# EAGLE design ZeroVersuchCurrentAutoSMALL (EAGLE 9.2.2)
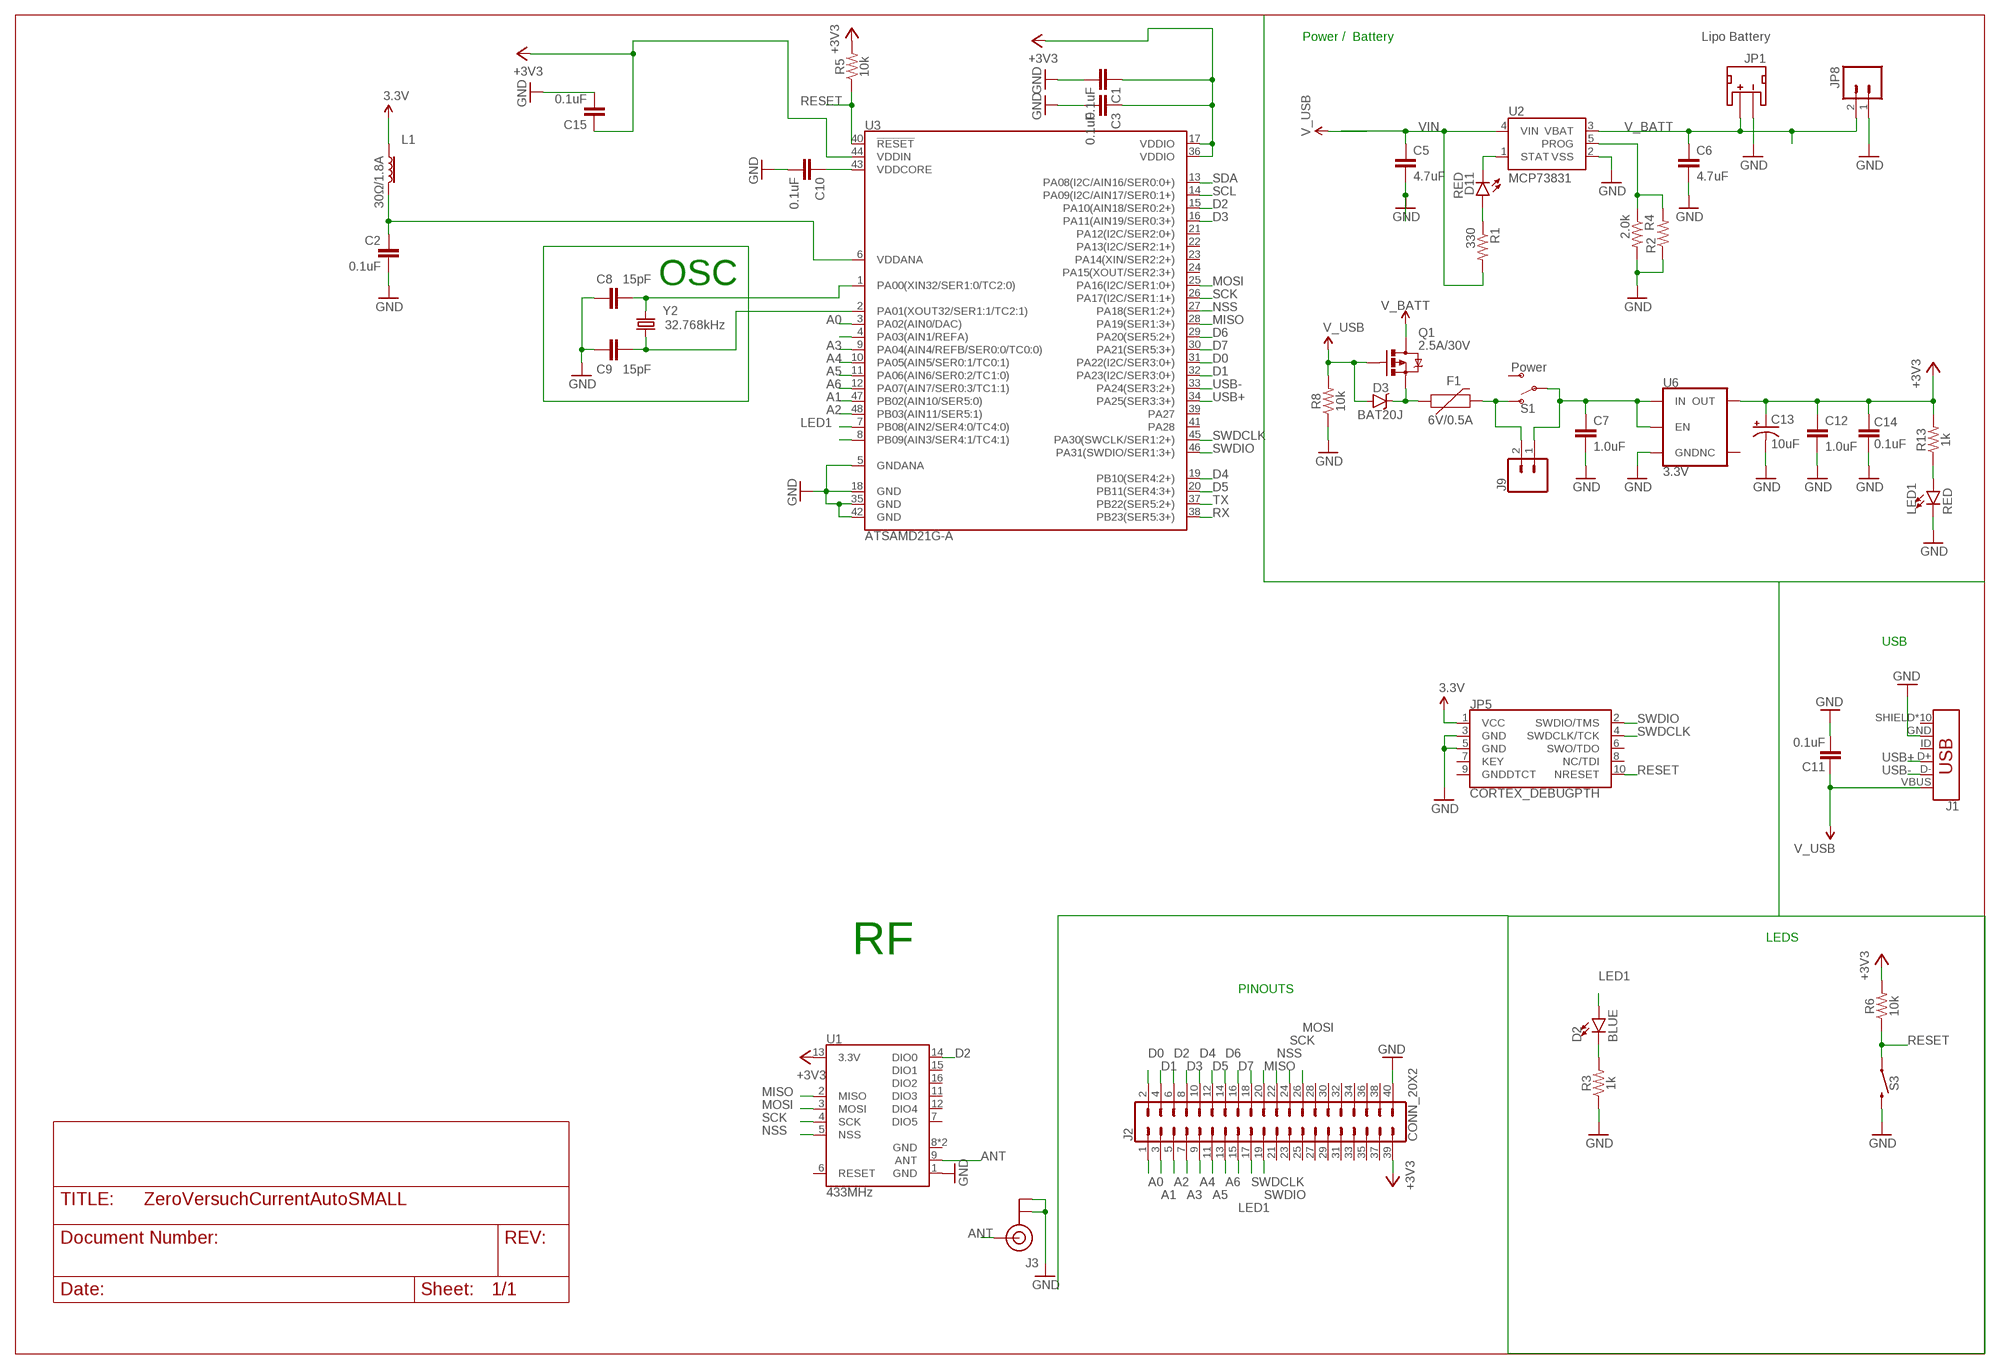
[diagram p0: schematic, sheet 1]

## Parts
C1  0.1uF  0.1UF-KIT-EZ-50V-20%  [CAP-PTH-SMALL-KIT]
C2  0.1uF  0.1UF-KIT-EZ-50V-20%  [CAP-PTH-SMALL-KIT]
C3  0.1uF  0.1UF-KIT-EZ-50V-20%  [CAP-PTH-SMALL-KIT]
C5  4.7uF  4.7UF-1206-16V-(+80/-20%)  [1206]
C6  4.7uF  4.7UF-1206-16V-(+80/-20%)  [1206]
C7  1.0uF  1.0UF-0603-16V-10%  [0603]
C8  15pF  15PF-0603-50V-5%  [0603]
C9  15pF  15PF-0603-50V-5%  [0603]
C10  0.1uF  0.1UF-KIT-EZ-50V-20%  [CAP-PTH-SMALL-KIT]
C11  0.1uF  0.1UF-KIT-EZ-50V-20%  [CAP-PTH-SMALL-KIT]
C12  1.0uF  1.0UF-0603-16V-10%  [0603]
C13  10uF  10UF-POLAR-RADIAL-2.5MM-KIT-25V-20%  [CPOL-RADIAL-2.5MM-5MM-KIT]
C14  0.1uF  0.1UF-KIT-EZ-50V-20%  [CAP-PTH-SMALL-KIT]
C15  0.1uF  0.1UF-KIT-EZ-50V-20%  [CAP-PTH-SMALL-KIT]
D2  BLUE  LED-BLUE1206  [LED-1206]
D3  BAT20J  DIODE-SCHOTTKY-BAT20J  [SOD-323]
D11  RED  LED-RED1206  [LED-1206]
F1  6V/0.5A  PPTC_HALF-AMP  [1206]
J1  USB_MICRO-B_HALF_PTH_MILL  [USB-MICROB-PTH-MILL]
J2  CONN_20X2  [2X20]
J3  U.FL  [U.FL]
J9  External On/Off  CONN_021X02_NO_SILK  [1X02_NO_SILK]
JP1  JST  JST_2MM_MALE  [JST-2-SMD@1]
JP5  CORTEX_DEBUGPTH  [2X5-PTH-1.27MM]
JP8  M02PTH  [1X02@1]
L1  30Ω/1.8A  FERRITE_BEAD-0603  [0603]
LED1  RED  LED-RED1206  [LED-1206]
Q1  2.5A/30V  MOSFET-PCHANNELDMG2307L  [SOT23-3]
R1  330  330OHM-HORIZ-1/10W-5%  [AXIAL-0.3]
R2  RESISTORPTH-1/4W-VERT-KIT  [AXIAL-0.1EZ]
R3  1k  1KOHM-HORIZ-1/4W-5%  [AXIAL-0.3]
R4  2.0k  2.0KOHM1/10W5%(0603)  [0603-RES]
R5  10k  10KOHM-HORIZ-1/4W-5%  [AXIAL-0.3]
R6  10k  10KOHM-HORIZ-1/4W-5%  [AXIAL-0.3]
R8  10k  10KOHM-HORIZ-1/4W-5%  [AXIAL-0.3]
R13  1k  1KOHM-HORIZ-1/4W-5%  [AXIAL-0.3]
S1  Power  SWITCH-SPDT-SMD-RIGHT-ANGLE  [SWITCH_SPST_SMD_A]
S3  MOMENTARY-SWITCH-SPST-SMD-RIGHT-ANGLE  [TACTILE_SWITCH_SMD_RIGHT_ANGLE]
U1  433MHz  RFM69HCW-433  [RFM69HCW-XXXS2]
U2  MCP73831  [SOT23-5]
U3  ATSAMD21G-A  [TQFP-48]
U6  3.3V  V_REG_AP2112K-3.3V  [SOT23-5]
Y2  32.768kHz  CRYSTAL-32.768KHZSMD-3.2X1.5  [CRYSTAL-SMD-3.2X1.5MM]

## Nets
3.3V [vcc]: JP5.1(VCC) L1.1
+3V3: C1.1 C3.1 C12.1 C13.1(+) C14.2 C15.1 J2.39 R5.P$2 R6.P$2 R13.P$2 U1.13(3.3V) U3.17(VDDIO) U3.36(VDDIO) U3.44(VDDIN) U6.5(OUT)
A0: J2.1 U3.3(PA02(AIN0/DAC))
A1: J2.3 U3.47(PB02(AIN10/SER5:0))
A2: J2.5 U3.48(PB03(AIN11/SER5:1))
A3: J2.7 U3.9(PA04(AIN4/REFB/SER0:0/TC0:0))
A4: J2.9 U3.10(PA05(AIN5/SER0:1/TC0:1))
A5: J2.11 U3.11(PA06(AIN6/SER0:2/TC1:0))
A6: J2.13 U3.12(PA07(AIN7/SER0:3/TC1:1))
ANT: J3.FEED(SIGNAL) U1.9(ANT)
D0: J2.2 U3.31(PA22(I2C/SER3:0+))
D1: J2.4 U3.32(PA23(I2C/SER3:0+))
D2: J2.6 U1.14(DIO0) U3.15(PA10(AIN18/SER0:2+))
D3: J2.8 U3.16(PA11(AIN19/SER0:3+))
D4: J2.10 U3.19(PB10(SER4:2+))
D5: J2.12 U3.20(PB11(SER4:3+))
D6: J2.14 U3.29(PA20(SER5:2+))
D7: J2.16 U3.30(PA21(SER5:3+))
GND: C1.2 C2.2 C3.2 C5.2 C6.2 C7.2 C8.1 C9.1 C10.2 C11.1 C12.2 C13.2(-) C14.1 C15.2 J1.GND J2.40 J3.1(GND) J3.2(GND) JP1.1(-) JP5.3(GND) JP5.5(GND) JP8.1 LED1.C R2.P$1 R3.P$1 R4.2 R8.P$1 S3.2 U1.1(GND) U2.2(VSS) U3.5(GNDANA) U3.18(GND) U3.35(GND) U3.42(GND) U6.2(GND)
LED1: D2.A J2.15 U3.7(PB08(AIN2/SER4:0/TC4:0))
MISO: J2.20 U1.2(MISO) U3.28(PA19(SER1:3+))
MOSI: J2.26 U1.3(MOSI) U3.25(PA16(I2C/SER1:0+))
N$1: D2.C R3.P$2
N$2: C10.1 U3.43(VDDCORE)
N$4: D11.A R1.P$1
N$8: C7.1 J9.1 S1.2(P) U6.1(IN) U6.3(EN)
N$9: F1.2 J9.2 S1.1(O)
N$10: C8.2 U3.1(PA00(XIN32/SER1:0/TC2:0)) Y2.P$2
N$11: C9.2 U3.2(PA01(XOUT32/SER1:1/TC2:1)) Y2.P$1
N$14: U3.4(PA03(AIN1/REFA))
N$15: J2.18
N$22: U3.8(PB09(AIN3/SER4:1/TC4:1))
N$38: LED1.A R13.P$1
NSS: J2.22 U1.5(NSS) U3.27(PA18(SER1:2+))
PROG: R2.P$2 R4.1 U2.5(PROG)
RAW [vcc]: D3.C F1.1 Q1.2(S)
RESET: JP5.10(NRESET) R5.P$1 R6.P$1 S3.1 U3.40(!RESET!)
RX: U3.38(PB23(SER5:3+))
SCK: J2.24 U1.4(SCK) U3.26(PA17(I2C/SER1:1+))
SCL: U3.14(PA09(I2C/AIN17/SER0:1+))
SDA: U3.13(PA08(I2C/AIN16/SER0:0+))
STAT: D11.C U2.1(STAT)
SWDCLK: J2.17 JP5.4(SWDCLK/TCK) U3.45(PA30(SWCLK/SER1:2+))
SWDIO: J2.19 JP5.2(SWDIO/TMS) U3.46(PA31(SWDIO/SER1:3+))
TX: U3.37(PB22(SER5:2+))
USB+: J1.D+ U3.34(PA25(SER3:3+))
USB-: J1.D- U3.33(PA24(SER3:2+))
V_BATT: C6.1 JP1.2(+) JP8.2 Q1.3(D) U2.3(VBAT)
V_USB: C11.2 D3.A J1.VBUS Q1.1(G) R8.P$2
VDDANA: C2.1 L1.2 U3.6(VDDANA)
VIN: C5.1 R1.P$2 U2.4(VIN)
Unconnected: J1.ID J1.SHIELD J1.SHIELD2(SHIELD) J1.SHIELD3(SHIELD) J1.SHIELD4(SHIELD) J1.SHIELD5(SHIELD) J1.SHIELD6(SHIELD) J1.SHIELD7(SHIELD) J1.SHIELD8(SHIELD) J1.SHIELD9(SHIELD) J1.SHIELD10(SHIELD) J2.21 J2.23 J2.25 J2.27 J2.28 J2.29 J2.30 J2.31 J2.32 J2.33 J2.34 J2.35 J2.36 J2.37 J2.38 JP1.NC1(PAD1) JP1.NC2(PAD2) JP5.6(SWO/TDO) JP5.7(KEY) JP5.8(NC/TDI) JP5.9(GNDDTCT) S1.3(S) U1.6(RESET) U1.7(DIO5) U1.11(DIO3) U1.12(DIO4) U1.15(DIO1) U1.16(DIO2) U3.21(PA12(I2C/SER2:0+)) U3.22(PA13(I2C/SER2:1+)) U3.23(PA14(XIN/SER2:2+)) U3.24(PA15(XOUT/SER2:3+)) U3.39(PA27) U3.41(PA28) U6.4(NC)

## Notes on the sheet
- Power /  Battery | Lipo Battery
- OSC
- USB
- LEDS
- RF
- PINOUTS

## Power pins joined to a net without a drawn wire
GND: U1.8(GND) U1.10(GND)

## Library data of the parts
C1-C3 C10 C11 C14 C15 = SparkFun-Capacitors:0.1UF: 0.1µF ceramic capacitors; PROD_ID: CAP-08370
C5 C6 = SparkFun-Capacitors:4.7UF: 4.7µF ceramic capacitors; PROD_ID: CAP-10300
C7 C12 = SparkFun-Capacitors:1.0UF: 1µF ceramic capacitors; PROD_ID: CAP-00868
C8 C9 = SparkFun-Capacitors:15PF: 15pF ceramic capacitors; PROD_ID: CAP-07881
C13 = SparkFun-Capacitors:10UF-POLAR: 10.0µF polarized capacitors; PROD_ID: CAP-08440
D2 = SparkFun-LED:LED-BLUE: Blue SMD LED; PROD_ID: DIO-09911
D3 = SparkFun-DiscreteSemi:DIODE-SCHOTTKY: Schottky diodes in SFE's production catalog; PROD_ID: DIO-11623
D11 LED1 = SparkFun-LED:LED-RED: Red SMD LED; PROD_ID: DIO-09912
F1 = SparkFun-Fuses:PPTC: Resettable Fuse PPTC; PROD_ID: RES-08585
J1 = SparkFun-Connectors:USB_MICRO-B: USB Type Micro-B Connector Male/female and PTH/SMT variants SparkFun Products: SparkFun microB USB Breakout SparkFun USB microB Plug Breakout SparkFun ESP8266 Thing; PROD_ID: CONN-13711
J2 = SparkFun-Connectors:CONN_20X2: Multi connection point. Often used as Generic Header-pin footprint for 0.1 inch spaced/style header connections On any of the 0.1 inch spaced packages, you can populate with these: Break Away Headers - Straight (PRT-00116) Break Away Male Headers - Right Angle (PRT-00553) Female Headers (PRT-00115)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
J3 = SparkFun-Connectors:U.FL: SMD Antenna Connector - U.FL 2mm height, 3.0mm x 3.0mm receptacle size. SparkFun Products: SparkFun WiFi Shield - ESP8266 SparkFun ESP8266 Thing SparkFun MiniGen - Pro Mini Signal Generator Shield; PROD_ID: CONN-09193; SF_ID: WRL-09144
J9 = SparkFun-Connectors:CONN_02: Multi connection point. Often used as Generic Header-pin footprint for 0.1 inch spaced/style header connections
JP1 = SparkFun-Connectors:JST_2MM_MALE: Mates to single-cell LiPo batteries. CONN-08352; PROD_ID: CONN-08352
JP5 = samd21-temp:CORTEX_DEBUG: Cortex Debug Connector Datasheet
JP8 = SparkFun-Connectors:M02: Standard 2-pin 0.1" header. Use with
L1 = SparkFun-Coils:FERRITE_BEAD: Ferrite Bead (blocks, cores, rings, chokes, etc.); PROD_ID: NDUC-07859
Q1 = SparkFun-DiscreteSemi:MOSFET-PCHANNEL: Generic PMOSFET IRLML2244 - TRANS-11153 (SOT-23 -20V -4.3A) (1.Gate 2.Source 3.Drain) FQP27P06 - COM-10349 (TO-220 -60V -27A) (1.Gate 2.Source 3.Drain); PROD_ID: TRANS-11308
R1 = SparkFun-Resistors:330OHM: 330Ω resistor; PROD_ID: RES-8371
R2 = SparkFun-Resistors:RESISTOR: Resistor
R3 R13 = SparkFun-Resistors:1KOHM: 1kΩ resistor; PROD_ID: RES-08380
R4 = SparkFun-Resistors:2.0KOHM1/10W5%(0603): RES-08296; PROD_ID: RES-08296
R5 R6 R8 = SparkFun-Resistors:10KOHM: 10kΩ resistor; PROD_ID: RES-09435
S1 = SparkFun-Switches:SWITCH-SPDT: Single Pole, Double Throw (SPDT) Switch Single-pole, double-throw (SPDT) switch. Variant Overview SMD-AYZ0202 Surface Mount DPDT Switch (COM-00597) Used on e.g. LilyPad Arduino USB - ATmega32U4 Board PTH-11.6X4.0MM SPDT Mini Power Switch (COM-00102) Used on e.g. SparkFun Simon Says - Through-Hole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; PROD_ID: SWCH-10651; SF_SKU: COM-10860
S3 = SparkFun-Switches:MOMENTARY-SWITCH-SPST: Momentary Switch (Pushbutton) - SPST; PROD_ID: COMP-12265
U1 = SparkFun-RF:RFM69H: Hope RF RFM69H ISM Transceiver Module The RFM69H is a transceiver module capable of operation over a wide frequency range, including the 315,433,868 and 915MHz license-free ISM (Industry Scientific and Medical) frequency bands. All major RF communication parameters are programmable and most of them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; PROD_ID: IC-12053
U2 = SparkFun-PowerIC:MCP73831: Miniature single cell, fully integrated Li-Ion, Li-polymer charge management controller http://ww1.microchip.com/downloads/en/DeviceDoc/21984a.pdf IC-09995; PROD_ID: IC-09995
U3 = SparkFun-IC-Microcontroller:ATSAMD21G: Atmel SAMD21G SMART ARM-Based Microcontroller The Atmel ® | SMART ™ SAM D21 is a series of low-power microcontrollers using the 32-bit ARM ® Cortex ® -M0+ processor, and ranging from 32- to 64-pins with up to 256KB Flash and 32KB of SRAM. The SAM D21 devices operate at a maximum frequency of 48MHz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; PROD_ID: IC-13064
U6 = SparkFun-IC-Power:V_REG_AP2112: AP2112 - 600mA CMOS LDO Regulator w/ Enable The AP2112 is CMOS process low dropout linear regulator with enable function, the regulator delivers a guaranteed 600mA (min.) continuous load current. Features Output Voltage Accuracy: ±1.5% Output Current: 600mA (Min.) Foldback Short Current Protection: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; PROD_ID: VREG-12457
Y2 = SparkFun-Clocks:CRYSTAL-32.768KHZ: 32.768kHz Crystal; PROD_ID: XTAL-13062

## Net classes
0 default: width 0.01 mm, drill 0.02 mm, clearance 0.006 mm
1 vcc: width 0.01 mm, drill 0.02 mm, clearance 0.006 mm to class 0

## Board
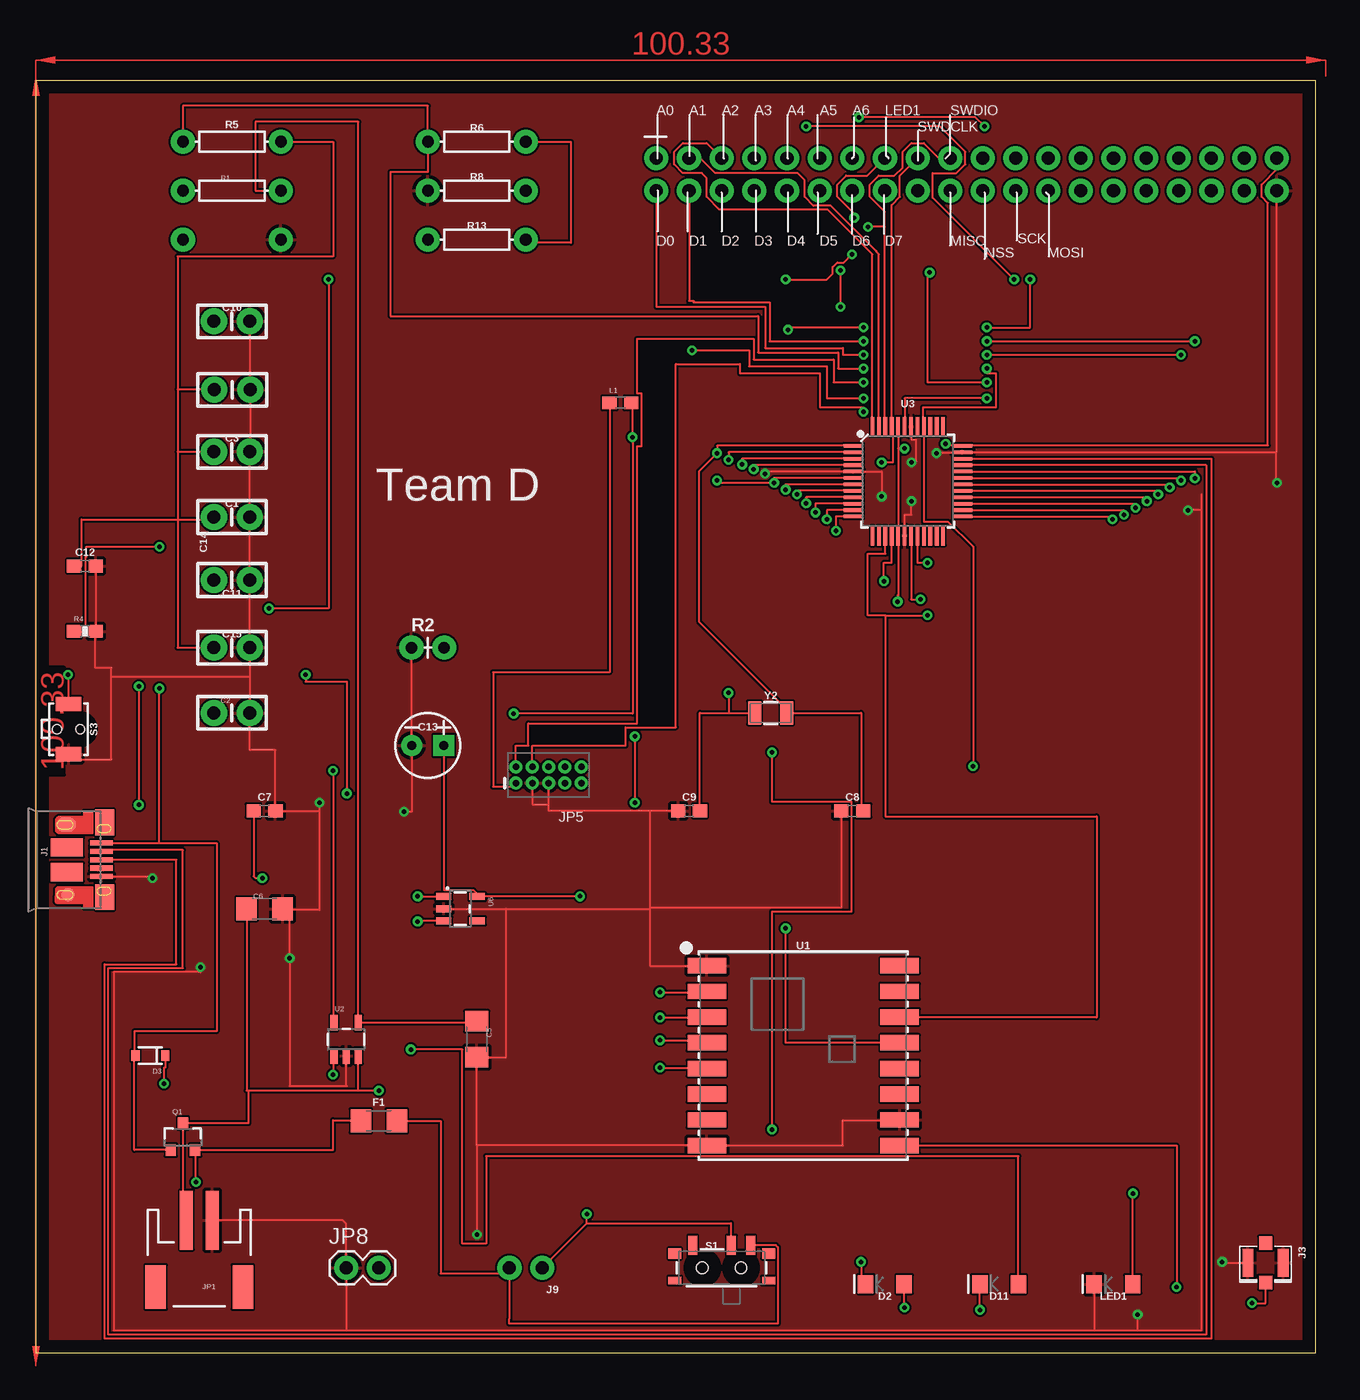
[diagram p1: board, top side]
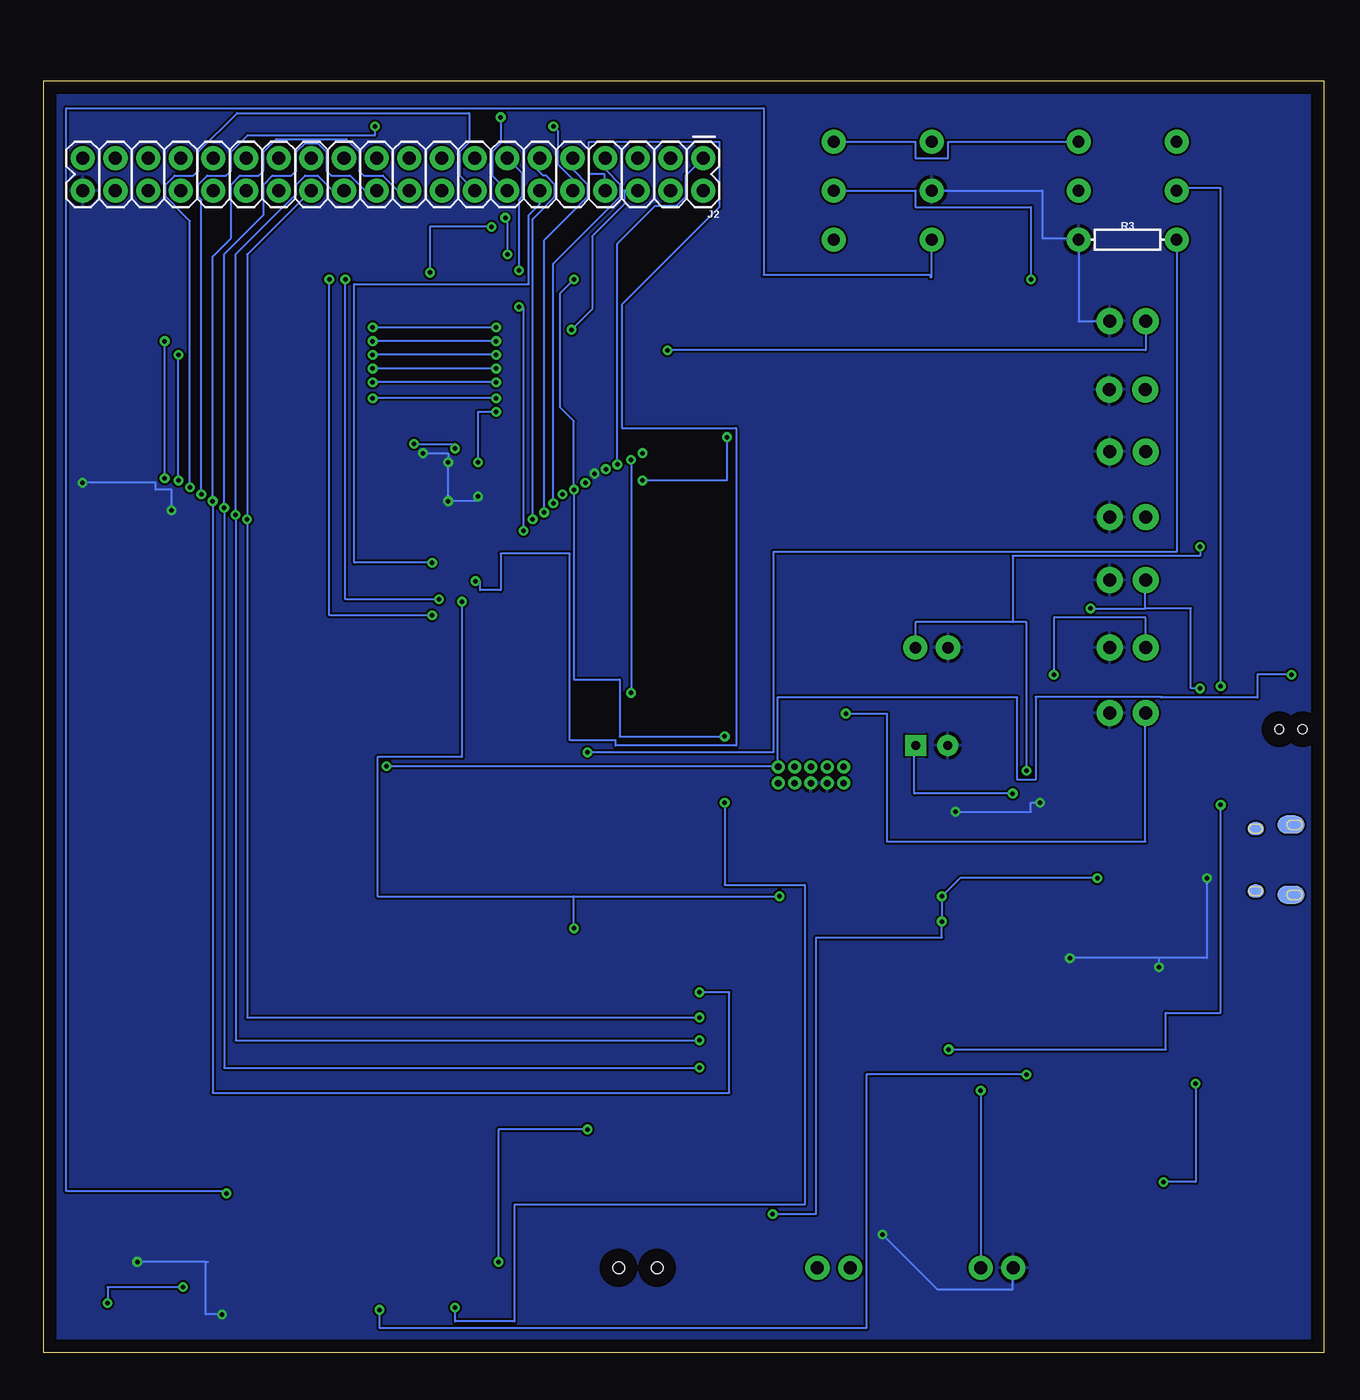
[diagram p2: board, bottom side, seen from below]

Size 99.55 x 98.98 mm. Coordinates in mm from the lower left corner, seen from the top.
Outline: 0,0 99.55,0 99.55,98.98 0,98.98 0,0
Copper layers (1*16): Top 0.035mm / dielectric 1.5mm / Bottom 0.035mm
Design rules "default": minimum track width 6mil, minimum drill 0.35mm, track to track 6mil, track to pad 6mil, pad to pad 6mil, via to via 6mil, smd to smd 6mil, copper to edge 40mil, drill to drill 6mil, minimum pad ring 10mil, minimum via ring 8mil, stop-mask expansion 4mil, vias tented up to drill 0mil, thermal gap 10mil

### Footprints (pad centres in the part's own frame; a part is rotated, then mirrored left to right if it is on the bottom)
CAP-PTH-SMALL-KIT = drill 1.016 pad 2.032: 1 -1.397,0; 2 1.397,0
1206 = smd 1.6 x 1.8: 1 -1.4,0; 2 1.4,0
0603 = smd 1.1 x 1: 1 -0.85,0; 2 0.85,0
CPOL-RADIAL-2.5MM-5MM-KIT = drill 0.7 pad 1.651 square: 1 1.25,0 | drill 0.7 pad 1.651: 2 -1.25,0
LED-1206 = smd 1.2 x 1.4: A -1.5,0; C 1.5,0
SOD-323 = smd 0.63 x 0.83: A 1.15,0; C -1.15,0
USB-MICROB-PTH-MILL = smd 0.4 x 1.75: D+ 0,0; D- -0.65,0; GND 1.3,0; ID 0.65,0; VBUS -1.3,0 | smd 2 x 1.46: SHIELD -2.9,0.275; SHIELD2 2.9,0.275 | smd 1.425 x 2.5: SHIELD3 -0.963,-2.675; SHIELD4 0.963,-2.675 | smd 1.4 x 2.1 bottom: SHIELD5 -2.731,-2.531; SHIELD7 2.729,-2.531 | smd 1 x 1: SHIELD6 2.7,-2.575 | smd 1.1 x 1.5: SHIELD8 -2.731,-2.731 | smd 1 x 1.3 bottom: SHIELD9 -2.43,0.195; SHIELD10 2.43,0.195
2X20 = drill 1.016 pad 1.88: 1 0,0; 2 0,2.54; 3 2.54,0; 4 2.54,2.54; 5 5.08,0; 6 5.08,2.54; 7 7.62,0; 8 7.62,2.54; 9 10.16,0; 10 10.16,2.54; 11 12.7,0; 12 12.7,2.54; 13 15.24,0; 14 15.24,2.54; 15 17.78,0; 16 17.78,2.54; 17 20.32,0; 18 20.32,2.54; 19 22.86,0; 20 22.86,2.54; 21 25.4,0; 22 25.4,2.54; 23 27.94,0; 24 27.94,2.54; 25 30.48,0; 26 30.48,2.54; 27 33.02,0; 28 33.02,2.54; 29 35.56,0; 30 35.56,2.54; 31 38.1,0; 32 38.1,2.54; 33 40.64,0; 34 40.64,2.54; 35 43.18,0; 36 43.18,2.54; 37 45.72,0; 38 45.72,2.54; 39 48.26,0; 40 48.26,2.54
U.FL = smd 2.2 x 0.85: 1 0,1.375; 2 0,-1.375 | smd 1.05 x 1: FEED 1.525,0; NC -1.525,0
1X02_NO_SILK = drill 1.016 pad 1.88: 1 0,0; 2 2.54,0
JST-2-SMD@1 = smd 1 x 4.6: 1 -1,-3.7; 2 1,-3.7 | smd 1.6 x 3.4: NC1 -3.4,1.5; NC2 3.4,1.5
2X5-PTH-1.27MM = drill 0.508 pad 1: 1 -2.54,-0.635; 2 -2.54,0.635; 3 -1.27,-0.635; 4 -1.27,0.635; 5 0,-0.635; 6 0,0.635; 7 1.27,-0.635; 8 1.27,0.635; 9 2.54,-0.635; 10 2.54,0.635
1X02@1 = drill 1.016 pad 1.88: 1 0,0; 2 2.54,0
SOT23-3 = smd 0.8 x 0.9: 1 -0.95,-1; 2 0.95,-1; 3 0,1.1
AXIAL-0.3 = drill 0.9 pad 1.88: P$1 -3.81,0; P$2 3.81,0
AXIAL-0.1EZ = drill 0.9 pad 1.88: P$1 0,0; P$2 2.54,0
0603-RES = smd 1.1 x 1: 1 -0.85,0; 2 0.85,0
SWITCH_SPST_SMD_A = smd 0.7 x 1.5: 1 -2.25,-1.75; 2 -0.75,-1.75; 3 2.25,-1.75 | smd 1 x 0.6: GND1 -3.65,1; GND3 3.65,1 | smd 1 x 0.8: GND2 -3.65,-1.1; GND4 3.65,-1.1 | hole 0.9: -1.5,0; 1.5,0
TACTILE_SWITCH_SMD_RIGHT_ANGLE = smd 1.1 x 2: 1 -1.95,0; 2 1.95,0 | hole 0.7: 0,0.9; 0,-0.9
RFM69HCW-XXXS2 = smd 3 x 1.2: 1 -7.5,7; 2 -7.5,5; 3 -7.5,3; 4 -7.5,1; 5 -7.5,-1; 6 -7.5,-3; 7 -7.5,-5; 8 -7.5,-7; 9 7.5,-7; 10 7.5,-5; 11 7.5,-3; 12 7.5,-1; 13 7.5,1; 14 7.5,3; 15 7.5,5; 16 7.5,7
SOT23-5 = smd 0.55 x 1.2: 1 -0.95,-1.3; 2 0,-1.3; 3 0.95,-1.3; 4 0.95,1.3; 5 -0.95,1.3
TQFP-48 = smd 1.5 x 0.28: 1 -4.25,2.75; 2 -4.25,2.25; 3 -4.25,1.75; 4 -4.25,1.25; 5 -4.25,0.75; 6 -4.25,0.25; 7 -4.25,-0.25; 8 -4.25,-0.75; 9 -4.25,-1.25; 10 -4.25,-1.75; 11 -4.25,-2.25; 12 -4.25,-2.75; 25 4.25,-2.75; 26 4.25,-2.25; 27 4.25,-1.75; 28 4.25,-1.25; 29 4.25,-0.75; 30 4.25,-0.25; 31 4.25,0.25; 32 4.25,0.75; 33 4.25,1.25; 34 4.25,1.75; 35 4.25,2.25; 36 4.25,2.75 | smd 0.28 x 1.5: 13 -2.75,-4.25; 14 -2.25,-4.25; 15 -1.75,-4.25; 16 -1.25,-4.25; 17 -0.75,-4.25; 18 -0.25,-4.25; 19 0.25,-4.25; 20 0.75,-4.25; 21 1.25,-4.25; 22 1.75,-4.25; 23 2.25,-4.25; 24 2.75,-4.25; 37 2.75,4.25; 38 2.25,4.25; 39 1.75,4.25; 40 1.25,4.25; 41 0.75,4.25; 42 0.25,4.25; 43 -0.25,4.25; 44 -0.75,4.25; 45 -1.25,4.25; 46 -1.75,4.25; 47 -2.25,4.25; 48 -2.75,4.25
CRYSTAL-SMD-3.2X1.5MM = smd 1 x 1.8: P$1 -1.25,0; P$2 1.25,0

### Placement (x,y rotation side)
C1  15.24,65.02 0 top
C2  15.24,49.78 0 top
C3  15.24,70.1 0 top
C5  34.29,24.38 270 top
C6  17.78,34.54 0 top
C7  17.78,42.16 0 top
C8  63.5,42.16 0 top
C9  50.8,42.16 0 top
C10  15.24,80.26 0 top
C11  15.24,60.12 180 top
C12  3.81,61.21 0 top
C13  30.48,47.24 0 top
C14  15.27,74.93 180 top
C15  15.24,54.86 0 top
D2  66.04,5.33 180 top
D3  8.89,23.11 180 top
D11  74.93,5.33 180 top
F1  26.67,18.03 0 top
J1  5.08,38.35 270 top
J2  48.26,92.96 180 bottom
J3  95.66,6.98 270 top
J9  39.37,6.6 180 top
JP1  12.7,6.6 180 top
JP5  39.88,44.96 0 top
JP8  24.13,6.6 0 top
L1  45.47,73.91 0 top
LED1  83.82,5.33 180 top
Q1  11.43,16.76 0 top
R1  15.24,90.42 0 top
R2  29.21,54.86 0 top
R3  15.24,86.61 0 bottom
R4  3.81,56.13 0 top
R5  15.24,94.23 0 top
R6  34.29,94.23 0 top
R8  34.29,90.42 0 top
R13  34.29,86.61 0 top
S1  53.34,6.6 180 top
S3  2.54,48.51 270 top
U1  59.69,23.11 0 top
U2  24.13,24.38 0 top
U3  67.82,67.82 0 top
U6  33.02,34.54 270 top
Y2  57.15,49.78 0 top

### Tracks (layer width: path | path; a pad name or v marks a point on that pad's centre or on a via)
3.3V
  Top 0.152: L1.1 44.62,52.93 35.56,52.93 35.56,44.04 37.34,44.04 JP5.1
+3V3  (via drill 0.35)
  Top 0.152: U3.44 67.07,70.36 | 67.07,70.36 U3.17 67.07,58.93 67.03,58.93 v67.03,58.45 | J2.39 96.52,92.08 95.35,90.91 95.35,89.94 95.83,89.46 95.83,70.61 72.07,70.61 U3.36 70.76,70.57 v70.76,70.71 | R5.P$2 23.11,94.23 23.11,85.29 11.02,85.29 11.02,74.98 | 11.02,70.1 C3.1 | 11.02,74.98 11.02,70.1 | 11.02,70.1 11.02,64.85 | 11.02,64.85 11.02,54.86 C15.1 | 11.02,64.85 13.84,64.85 C1.1 | 11.02,74.98 13.87,74.98 C14.2 | C13.1 31.73,36 34.02,36 34.49,35.52 34.49,35.51 | C12.1 3.56,61.21 3.56,64.85 11.02,64.85 | U1.13 58.32,24.11 v58.32,33.02 | R6.P$2 41.6,94.23 41.6,86.36 38.1,86.36 R13.P$2 | v20.98,52.76 20.98,52.22 24.18,52.22 v24.18,43.51 | 67.07,70.36 v67.56,70.36 | U6.5 34.34,35.51 34.49,35.51 | v42.32,35.51 34.49,35.51
  Bottom 0.152: v58.32,33.02 58.32,35.51 | 58.32,35.51 v42.32,35.51 | R6.P$2 31.75,94.23 31.75,92.96 29.21,92.96 29.21,94.23 R5.P$2 | v67.03,58.45 67.03,46.35 73.61,46.35 73.61,35.51 58.32,35.51 | C15.1 13.84,57.2 20.98,57.2 v20.98,52.76 | v24.18,43.51 31.83,43.51 31.83,47.24 C13.1 | v70.76,70.71 67.56,70.71 v67.56,70.36
A0  (via drill 0.35)
  Top 0.152: U3.3 54.94,69.57 v54.94,69.11
  Bottom 0.152: v54.94,69.11 54.94,86.28 51.97,89.26 50.32,89.26 49.63,89.94 49.63,91.59 J2.1
A1
  Top 0.152: U3.47 65.57,85.47 65.37,85.67 65.37,85.72 61.84,89.26 60.48,89.26 59.79,89.94 59.79,91.25 59.24,91.8 52.86,91.8 51.69,92.96 J2.3
A2
  Top 0.152: U3.48 65.07,85.47 61.59,88.95 53.16,88.95 52.17,89.94 52.17,91.41 51.79,91.8 50.32,91.8 49.63,92.48 49.63,93.45 50.32,94.13 52.17,94.13 J2.5
A3  (via drill 0.35)
  Top 0.152: U3.9 59.92,66.57 v59.92,66.09
  Bottom 0.152: v59.92,66.09 59.92,84.73 54.71,89.94 54.71,90.91 55.88,92.08 J2.7
A4  (via drill 0.35)
  Top 0.152: U3.10 60.63,66.07 v60.63,65.38
  Bottom 0.152: v60.63,65.38 60.63,86.56 57.25,89.94 57.25,90.91 58.42,92.08 J2.9
A5  (via drill 0.35)
  Top 0.152: U3.11 61.52,65.56 v61.52,64.85
  Bottom 0.152: J2.11 61.52,92.41 60.71,91.59 60.48,91.59 59.79,90.91 59.79,89.94 61.52,88.21 v61.52,64.85
A6  (via drill 0.35)
  Top 0.152: U3.12 62.23,65.07 v62.23,63.96 | v62.59,81.38 v62.59,84.23
  Bottom 0.152: v62.23,63.96 62.23,81.38 v62.59,81.38 | v62.59,84.23 62.59,89.69 62.33,89.94 62.33,91.8 J2.13
ANT  (via drill 0.35)
  Top 0.152: U1.9 88.72,16.11 v88.72,5.11 | v94.59,3.86 95.66,3.86 J3.FEED
  Bottom 0.152: v88.72,5.11 94.59,5.11 v94.59,3.86
D0  (via drill 0.35)
  Top 0.152: v89.08,67.87 89.08,68.07 U3.31 | J2.2 48.26,81.38 56.72,81.38 56.72,78.18 62.76,78.18 62.76,77.65 v64.36,77.65 | v73.97,77.65 v89.08,77.65
  Bottom 0.152: v89.08,67.87 v89.08,77.65 | v64.36,77.65 v73.97,77.65 74.14,77.65
D1  (via drill 0.35)
  Top 0.152: U3.32 90.14,68.57 v90.14,68.05 | J2.4 50.8,81.86 51.16,81.86 51.16,81.74 57.07,81.74 57.07,78.72 v64.36,78.72 | v73.97,78.72 v90.14,78.72
  Bottom 0.152: v90.14,68.05 v90.14,78.72 | v64.36,78.72 v73.97,78.72 74.14,78.72
D2  (via drill 0.35)
  Top 0.152: 66.07,57.38 66.07,41.73 82.5,41.73 82.5,26.09 67.19,26.09 U1.14 | 66.07,57.38 v69.34,57.38 | v64.36,79.78 58.67,79.78 v58.5,79.6 | v73.97,79.78 77.34,79.78 v77.34,83.52 | 66.07,57.38 64.72,57.38 64.72,62.18 66.07,62.18 U3.15
  Bottom 0.152: v69.34,57.38 77.34,57.38 v77.34,83.52 | J2.6 54.41,90.42 54.41,89.36 56.9,86.87 56.9,81.2 v58.5,79.6 | v64.36,79.78 v73.97,79.78
D3  (via drill 0.35)
  Top 0.152: v65.96,60.05 65.96,61.47 66.57,61.47 U3.16
  Bottom 0.152: J2.8 55.93,90.47 55.93,91.69 57.15,91.69 57.15,94.23 46.99,94.23 46.99,89.15 54.58,81.56 54.58,71.95 45.7,71.95 45.7,47.25 55.07,47.25 55.07,47.65 58.62,47.65 58.62,62.18 64.01,62.18 64.01,59.34 65.61,59.34 65.61,60.04 v65.96,60.04 v65.96,60.05
D4  (via drill 0.35)
  Top 0.152: U3.19 68.07,58.62 v68.81,58.62 | v76.1,83.52 69.75,89.86 69.75,91.8 71.6,91.8 72.29,92.48 72.29,93.45 70.31,95.43 v59.92,95.43
  Bottom 0.152: v68.81,58.62 76.1,58.62 v76.1,83.52 | v59.92,95.43 59.59,95.1 59.59,92.48 58.42,91.31 J2.10
D5  (via drill 0.35)
  Top 0.152: U3.20 68.57,61.47 v69.34,61.47
  Bottom 0.152: v69.34,61.47 75.39,61.47 75.39,83.16 61.82,83.16 61.82,88.52 60.96,89.38 J2.12
D6  (via drill 0.35)
  Top 0.152: v87.3,66.8 87.3,67.07 U3.29 | v73.79,95.43 73.08,96.14 v64.01,96.14
  Bottom 0.152: v87.3,66.8 87.3,89.71 87.53,89.94 87.53,90.91 86.84,91.59 85.37,91.59 84.99,91.97 84.99,93.45 83.69,94.74 73.79,94.74 v73.79,95.43 | v64.01,96.14 64.01,94.11 64.67,93.45 64.67,91.59 J2.14
D7  (via drill 0.35)
  Top 0.152: U3.30 88.19,67.57 v88.19,67.33
  Bottom 0.152: v88.19,67.33 88.19,88.06 90.07,89.94 90.07,90.91 89.38,91.59 87.91,91.59 87.53,91.97 87.53,93.45 84.51,96.47 66.47,96.47 66.47,94.19 67.21,93.45 67.21,91.59 J2.16
GND  (via drill 0.35)
  Top 0.152: C9.1 47.75,42.16 | 47.75,42.16 47.75,34.62 | 47.75,34.62 47.75,34.54 | 47.75,34.54 47.75,30.11 U1.1 | JP5.3 38.61,42.67 39.88,42.67 | 39.88,42.67 JP5.5 | 47.75,42.16 39.88,42.16 39.88,42.67 | U6.2 31.83,34.54 | 31.83,34.54 36.58,34.54 | 36.58,34.54 47.75,34.54 | 34.29,16.11 U1.8 62.76,16.11 62.76,18.09 67.19,18.09 U1.10 | 34.29,16.11 C5.2 36.58,22.98 36.58,34.54 | 96.48,70.07 U3.35 72.07,70 v70.05,70 | 96.48,70.07 96.48,90.33 96.52,90.37 J2.40 | 22.05,42.16 C7.2 18.63,46.89 16.64,46.89 C2.2 16.64,52.58 | 22.05,42.16 22.05,34.44 19.74,34.44 | 19.74,34.44 19.18,34.44 C6.2 | 31.83,34.44 31.83,34.54 | R2.P$1 29.23,54.86 C13.2 29.23,42.09 v28.63,42.09 | v56.72,68.4 56.72,68.57 U3.5 63.57,68.58 65.79,68.58 v65.79,66.62 | S3.2 2.54,46.18 5.87,46.18 5.87,52.58 | 5.87,52.58 5.87,53.29 4.62,53.29 4.62,55.96 | 4.62,55.96 4.62,56.13 R4.2 | 16.64,52.58 C15.2 C11.1 C1.2 16.64,69.83 | 16.64,69.83 C3.2 | C10.2 16.66,80.26 C14.1 16.66,69.83 16.64,69.83 | C8.1 62.65,34.62 47.75,34.62 | 34.29,16.11 34.29,9.22 v34.31,9.2 | JP1.1 23.86,10.3 24.13,10.03 JP8.1 24.18,6.6 24.18,1.73 | C12.2 4.66,55.96 4.62,55.96 | 16.64,52.58 5.87,52.58 | J1.GND 9.07,37.05 v9.07,36.93 | 19.74,34.44 v19.74,30.71 19.74,20.75 24.13,20.75 | 24.18,20.75 24.13,20.75 | 24.13,20.75 U2.2 | v12.8,30 12.8,29.62 6.04,29.62 6.04,1.73 24.18,1.73 | 90.68,65.56 90.68,1.73 85.7,1.73 | 90.68,65.56 90.68,66.8 | 24.18,1.73 82.32,1.73 | 82.32,1.73 85.7,1.73 | 90.68,65.56 v89.61,65.56 | v96.55,67.69 96.48,67.69 96.48,70.07 | v22.05,42.8 22.05,42.16 | LED1.C 82.32,1.73 | 85.7,1.73 v85.7,2.97 | v92.28,7.06 92.28,6.98 J3.2 | U3.18 67.57,65.2 68.1,65.2 v68.1,66.27 | U3.42 68.1,72.07 68.1,71.07 68.45,71.07 68.45,69.29 v68.1,69.29
  Bottom 0.152: R8.P$1 21.87,90.42 21.87,86.72 19.05,86.72 R3.P$1 19.05,80.26 C10.2 | v34.31,9.2 30.05,4.93 24.18,4.93 24.18,6.55 JP8.1 | v9.07,36.93 9.07,30.71 12.8,30.71 | 12.8,30.71 v19.74,30.71 | 12.8,30.71 v12.8,30 | v89.61,65.56 89.61,67.16 90.85,67.16 90.85,67.69 v96.55,67.69 | v28.63,42.09 22.76,42.09 22.76,42.8 v22.05,42.8 | v85.7,2.97 86.94,2.97 86.94,7.06 | 86.94,7.06 86.77,7.06 | 86.94,7.06 v92.28,7.06 | v65.79,66.62 65.79,66.27 v68.1,66.27 v68.1,69.29 68.1,70 v70.05,70
  pour Top: 0,0 99.57,0 99.57,99.31 0,99.31
  pour Bottom: 0,0.51 99.57,0.51 99.57,98.81 0,98.81
LED1  (via drill 0.35)
  Top 0.152: 63.57,67.51 U3.7 58.32,67.57 v58.32,67.16 | v46.58,47.95 v46.58,42.8 46.76,42.8 | v58.32,83.52 61.52,83.52 61.98,83.97 61.98,84.48 62.33,84.83 62.84,84.83 v63.48,85.47 | v63.65,88.32 63.65,88.62 62.33,89.94 62.33,90.91 63.02,91.59 64.67,91.59 J2.15 | v67.56,3.5 67.54,3.53 D2.A
  Bottom 0.152: v46.58,47.95 54.76,47.95 54.76,52.4 58.32,52.4 v58.32,67.16 58.32,72.49 59.38,73.56 59.38,82.45 v58.32,83.52 | v46.58,42.8 46.58,36.4 40.36,36.4 40.36,11.51 62.94,11.51 62.94,2.44 67.56,2.44 v67.56,3.5 | v63.48,85.47 63.48,88.14 v63.65,88.32
MISO  (via drill 0.35)
  Top 0.152: U3.28 86.41,66.57 v86.41,66.27 | v48.54,28.04 52.19,28.04 U1.2
  Bottom 0.152: v48.54,28.04 46.23,28.04 46.23,20.22 86.41,20.22 v86.41,66.27 86.41,85.29 84.99,86.72 84.99,90.91 84.3,91.59 82.83,91.59 82.45,91.97 82.45,93.45 81.46,94.44 76.02,94.44 75.03,93.45 75.03,91.97 74.65,91.59 73.18,91.59 72.01,90.42 J2.20
MOSI  (via drill 0.35)
  Top 0.152: U3.25 83.74,65.07 v83.74,64.85 | v48.54,26.09 52.19,26.09 U1.3
  Bottom 0.152: v48.54,26.09 83.74,26.09 v83.74,64.85 83.74,85.47 83.69,85.47 J2.26
N$1  (via drill 0.35)
  Top 0.152: v57.25,17.37 57.25,34.31 63.43,34.31 63.43,42.89 57.25,42.89 v57.25,46.71 | v64.19,7.06 64.19,5.33 D2.C
  Bottom 0.152: R3.P$2 11.43,62.31 42.8,62.31 42.8,46.71 v57.25,46.71 | v57.25,17.37 64.19,17.37 v64.19,7.06
N$2  (via drill 0.35)
  Top 0.152: v51.03,78 55.47,78 55.47,76.76 61.52,76.76 61.52,74.27 v64.36,74.27 | v73.97,74.27 67.57,74.27 U3.43
  Bottom 0.152: C10.1 13.84,78 v51.03,78 | v64.36,74.27 v73.97,74.27 74.14,74.27
N$4  (via drill 0.35)
  Top 0.152: v29.16,23.6 33.16,23.6 33.16,8.49 35.02,8.49 35.02,15.29 76.43,15.29 D11.A | v8,51.87 v8,42.62
  Bottom 0.152: v29.16,23.6 12.27,23.6 12.27,26.44 8,26.44 v8,42.62 | v8,51.87 8,90.63 11.43,90.63 R1.P$1
N$8  (via drill 0.35)
  Top 0.152: C7.1 16.93,37.07 17.07,36.93 v17.6,36.93 | v29.69,35.51 29.71,35.49 U6.1 | J9.1 42.85,10.08 | 42.85,10.08 54.05,10.08 54.05,8.39 S1.2 | U6.3 29.69,33.59 v29.69,33.55 | 42.85,10.08 v42.85,10.79
  Bottom 0.152: v17.6,36.93 28.27,36.93 v29.69,35.51 v29.69,33.55 29.69,32.31 39.47,32.31 39.47,10.79 v42.85,10.79
N$9
  Top 0.152: F1.2 31.47,18.03 31.47,6.17 36.83,6.17 J9.2 36.83,2.64 36.8,2.62 36.8,2.26 57.72,2.26 57.72,8.2 57.56,8.35 S1.1
N$10  (via drill 0.35)
  Top 0.152: U3.1 52.98,70.57 v52.98,70 51.56,68.58 51.56,56.9 58.67,49.78 | Y2.P$2 58.67,49.78 | 58.67,49.78 64.19,49.78 64.19,42.16 C8.2
N$11  (via drill 0.35)
  Top 0.152: U3.2 53.87,70.07 v53.87,69.47 | C9.2 51.65,49.78 53.87,49.78 | 53.87,49.78 Y2.P$1 | v53.87,51.33 53.87,49.78
  Bottom 0.152: v53.87,69.47 v53.87,51.33
N$14  (via drill 0.35)
  Top 0.152: U3.4 55.83,69.07 v55.83,68.76
N$22  (via drill 0.35)
  Top 0.152: U3.8 59.21,67.07 v59.21,66.8
N$38  (via drill 0.35)
  Top 0.152: LED1.A 85.32,12.4 v85.34,12.4
  Bottom 0.152: v85.34,12.4 85.34,12.57 97.79,12.57 97.79,96.85 43.56,96.85 43.56,83.87 30.58,83.87 30.58,83.69 30.48,83.69 R13.P$1
NSS  (via drill 0.35)
  Top 0.152: U3.27 85.52,66.07 v85.52,65.73 | v48.54,22.17 52.19,22.17 U1.5
  Bottom 0.152: v48.54,22.17 85.52,22.17 v85.52,65.73 85.52,85.47 82.45,88.54 82.45,90.91 81.76,91.59 80.29,91.59 79.91,91.97 79.91,93.45 79.22,94.13 78.26,94.13 77.57,93.45 77.57,91.97 77.19,91.59 75.72,91.59 74.55,90.42 J2.22
PROG  (via drill 0.35)
  Top 0.152: U2.5 23.18,45.35 v23.11,45.29 | R4.1 3.88,56.13 3.88,61.94 3.91,61.94 3.91,62.71 v9.6,62.71
  Bottom 0.152: v23.11,45.29 23.11,56.84 24.18,56.84 | R2.P$2 31.75,56.84 24.18,56.84 | v9.6,62.71 9.6,62 24.18,62 24.18,56.84
RAW  (via drill 0.35)
  Top 0.152: Q1.2 12.45,15.76 | 12.45,15.76 23.11,15.76 23.11,18.09 25.27,18.09 F1.1 | D3.C 10.04,22.17 9.96,22.17 v9.96,20.93 | v12.45,13.28 12.45,15.76
  Bottom 0.152: v12.45,13.28 9.96,13.28 v9.96,20.93
RESET  (via drill 0.35)
  Top 0.152: R5.P$1 11.43,97.03 30.48,97.03 R6.P$1 30.48,91.87 27.56,91.87 27.56,80.67 56.19,80.67 56.19,77.83 62.41,77.83 62.41,76.58 v64.36,76.58 | v72.9,45.64 72.9,62.71 70.94,64.67 69.07,64.67 U3.40 68.99,72.07 68.99,73.56 74.67,73.56 74.67,76.22 73.97,76.22 v73.97,76.58 | S3.1 2.54,52.76 v2.49,52.76
  Bottom 0.152: v72.9,45.64 42.49,45.64 | 42.49,45.64 42.42,45.64 JP5.10 | v2.49,52.76 5.16,52.76 5.16,50.98 12.6,50.98 12.6,51.03 22.41,51.03 22.41,44.58 23.82,44.58 23.82,50.98 42.49,50.98 42.49,45.64 | v64.36,76.58 v73.97,76.58
SCK  (via drill 0.35)
  Top 0.152: U3.26 84.63,65.57 v84.63,65.2 | v48.54,24.31 52.19,24.31 U1.4
  Bottom 0.152: v48.54,24.31 84.63,24.31 v84.63,65.2 84.63,85.47 80.85,89.26 80.8,89.26 79.91,90.14 79.91,90.91 79.22,91.59 78.26,91.59 77.09,90.42 J2.24
STAT  (via drill 0.35)
  Top 0.152: U2.1 23.11,23.08 v23.11,21.64 | v73.43,3.33 D11.C
  Bottom 0.152: v73.43,3.33 73.43,1.91 35.56,1.91 35.56,21.64 v23.11,21.64
SWDCLK  (via drill 0.35)
  Top 0.152: JP5.4 38.61,47.24 45.88,47.24 45.88,48.66 49.78,48.66 49.78,76.94 54.76,76.94 54.76,76.22 60.98,76.22 60.98,73.56 64.36,73.56 v64.36,73.2 | J2.17 67.21,91.59 67.21,89.94 66.57,89.3 U3.45 66.57,71.6 66.67,71.6 66.67,69.29 v65.79,69.29
  Bottom 0.152: v64.36,73.2 65.79,73.2 v65.79,69.29
SWDIO  (via drill 0.35)
  Top 0.152: JP5.2 37.34,47.24 38.3,47.24 38.3,48.97 46.76,48.97 46.76,70.54 47.11,70.54 47.11,74.64 46.76,74.64 46.76,78.89 55.83,78.89 55.83,77.29 62.05,77.29 62.05,75.51 v64.36,75.51 | U3.46 66.04,72.07 66.04,87.61 | J2.19 70.23,92.96 69.06,94.13 68.1,94.13 67.41,93.45 67.41,92.23 66.78,91.59 65.56,91.59 64.87,90.91 64.87,89.94 66.04,88.77 66.04,87.61 | 66.04,87.61 v64.72,87.61 | v69.52,84.05 69.34,84.05 69.34,75.51 v73.97,75.51
  Bottom 0.152: v64.36,75.51 v73.97,75.51 | v64.72,87.61 69.52,87.61 v69.52,84.05
USB+
  Top 0.152: U3.34 91.44,69.57 91.44,1.09 5.33,1.09 5.33,30.23 10.92,30.23 10.92,38.35 J1.D+
USB-
  Top 0.152: U3.33 91.03,69.07 91.03,1.4 5.64,1.4 5.64,29.92 11.43,29.92 11.43,39.12 5.08,39.12 J1.D-
V_BATT  (via drill 0.35)
  Top 0.152: C6.1 16.38,20.4 16.54,20.4 | 25.08,20.4 U2.3 | 16.54,20.4 25.08,20.4 | 25.08,20.4 v26.67,20.4 | 16.54,20.4 16.54,17.86 Q1.3 11.43,10.3 JP1.2
  Bottom 0.152: v26.67,20.4 JP8.2
V_USB  (via drill 0.35)
  Top 0.152: v22.76,83.52 22.76,57.91 v18.14,57.91 | Q1.1 7.64,15.77 7.64,23.11 | J1.VBUS 9.6,39.65 | 9.6,39.65 v9.6,51.69 | 9.6,39.65 14.05,39.65 14.05,25.02 7.64,25.02 7.64,23.11 | 7.64,23.11 D3.A
  Bottom 0.152: R8.P$2 31.75,90.42 31.75,89.15 22.76,89.15 v22.76,83.52 | v18.14,57.91 13.87,57.91 | 13.87,57.91 13.87,60.12 C11.2 | v9.6,51.69 10.31,51.69 10.31,57.91 13.87,57.91
VDDANA  (via drill 0.35)
  Top 0.152: L1.2 46.41,73.91 v46.41,71.25 46.41,49.73 v37.16,49.73 | U3.6 57.43,68.07 v57.43,67.69 53.16,67.69 v52.98,67.87
  Bottom 0.152: v46.41,71.25 46.41,67.87 v52.98,67.87 | v37.16,49.73 33.96,49.73 33.96,39.78 13.87,39.78 13.87,49.78 C2.1
VIN
  Top 0.152: C5.1 34.19,25.68 U2.4 25.08,95.78 17.07,95.78 17.07,90.42 R1.P$2
(copper drawn outside any net)
  shapes: Top area x2

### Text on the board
tPlace: A0 | A1 | A2 | A3 | A4 | A5 | A6 | LED1 | SWDIO | SWDCLK | D0 | D1 | D2 | D3 | D4 | D5 | D6 | D7 | MISO | SCK | NSS | MOSI | Team D | 3.3V | GND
